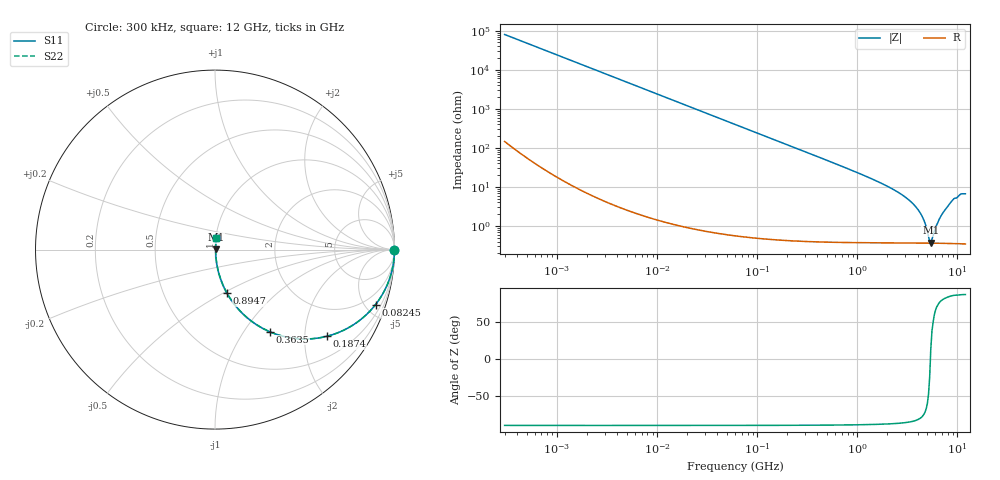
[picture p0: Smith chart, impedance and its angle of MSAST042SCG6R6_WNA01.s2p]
! MSAST042SCG6R6_WNA01  S-PARAMETER MODEL  ( General Type )
! Model Generated by TAIYO YUDEN Corporation (http://www.ty-top.com)
! Version 1.0
! TAIYO YUDEN Control No. 150820
! Copyright(c) 2015 TAIYO YUDEN CO.,LTD. All Rights Reserved.
! Product Description (link to TY-COMPAS)
! https://ds.yuden.co.jp/TYCOMPAS/or/detail?pn=MSAST042SCG6R6BWNA01&u=M
! Products Name : Multilayer Ceramic Capacitors
! Characteristics :
!  Capacitance : 6.6 pF , Rated Voltage : 25V , TCC : CG / C0G
!  Case Size : 0.4 x 0.2 / 0.016 x 0.008 [mm/inch] , Thickness : 0.2 / 0.008 [mm/inch]
!  (Conditions: Temperature = 25 degC , DC Bias Current/Voltage = 0A / 0V)
! External Node Assignments :
!  1  o---| |---o  2
! GND o---------o GND
! Frequency Range : 0.3MHz  -  12000MHz  [ 401 STEP ]
# MHz S RI R 50
! Freq[MHz].  S11 Real  S11 Imag  S21 Real  S21 Imag  S12 Real  S12 Imag  S22 Real  S22 Imag
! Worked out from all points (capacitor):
!   401 points, 300 kHz to 12 GHz, reference 50 ohm
!   read as one part in series: C = 6.61 pF near 316.3 kHz
!   lowest |Z| = 376 mohm at 5.42 GHz (marker M1)
!   series resonance near 5.369 GHz, so ESL is about 130 pH
!   S11 on the Smith chart (normalised r, x): 300 kHz: open; 82.45 MHz: 1.01, -5.84; 187.4 MHz: 1.01, -2.57; 363.5 MHz: 1.01, -1.32; 894.7 MHz: 1.01, -0.52; 12 GHz: 1.01, +0.13
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0.3  1 -0.00125  3.82e-06 0.00125  3.82e-06 0.00125  1 -0.00125
1.769972  0.9999 -0.00735  5.84e-05 0.00735  5.84e-05 0.00735  0.9999 -0.00735
10.44266  0.9981 -0.0433  0.0019 0.0433  0.0019 0.0433  0.9981 -0.0433
27.10171  0.9874 -0.1112  0.0126 0.1112  0.0126 0.1112  0.9874 -0.1112
60  0.9412 -0.2345  0.0588 0.2345  0.0588 0.2345  0.9412 -0.2345
82.45425  0.8945 -0.3063  0.1055 0.3063  0.1055 0.3063  0.8945 -0.3063
187.4445  0.6216 -0.4833  0.3784 0.4833  0.3784 0.4833  0.6216 -0.4833
353.9943  0.3153 -0.4617  0.6847 0.4617  0.6847 0.4617  0.3153 -0.4617
363.4975  0.304 -0.457  0.696 0.457  0.696 0.457  0.304 -0.457
555.3718  0.1575 -0.3599  0.8425 0.3599  0.8425 0.3599  0.1575 -0.3599
894.6982  0.0671 -0.2431  0.9329 0.2431  0.9329 0.2431  0.0671 -0.2431
2088.533  0.0131 -0.0962  0.9869 0.0962  0.9869 0.0962  0.0131 -0.0962
3026.31  0.00659 -0.0538  0.9934 0.0538  0.9934 0.0538  0.00659 -0.0538
3944.255  0.00444 -0.0279  0.9956 0.0279  0.9956 0.0279  0.00444 -0.0279
4502.883  0.0039 -0.0158  0.9961 0.0158  0.9961 0.0158  0.0039 -0.0158
5140.631  0.00365 -0.00397  0.9964 0.00397  0.9964 0.00397  0.00365 -0.00397
5420.343  0.00363 0.000932  0.9964 -0.000932  0.9964 -0.000932  0.00363 0.000932
5565.855  0.00363 0.00282  0.9964 -0.00282  0.9964 -0.00282  0.00363 0.00282
6699.894  0.00385 0.0158  0.9962 -0.0158  0.9962 -0.0158  0.00385 0.0158
8064.993  0.00464 0.0327  0.9954 -0.0327  0.9954 -0.0327  0.00464 0.0327
10511.28  0.00732 0.0616  0.9927 -0.0616  0.9927 -0.0616  0.00732 0.0616
12000  0.00783 0.0659  0.9922 -0.0659  0.9922 -0.0659  0.00783 0.0659
